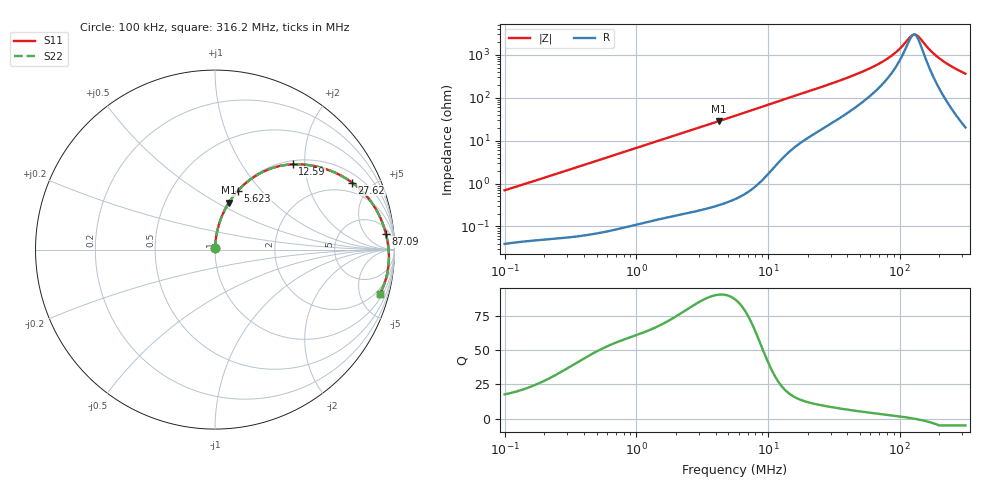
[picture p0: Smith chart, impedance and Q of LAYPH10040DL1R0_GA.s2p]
! LAYPH10040DL1R0_GA  S-PARAMETER MODEL  ( General Type )
! Model Generated by TAIYO YUDEN Corporation (http://www.ty-top.com)
! Version 1.0
! TAIYO YUDEN Control No. 180920NI43SB-FBB
! Copyright(c) 2018 TAIYO YUDEN CO.,LTD. All Rights Reserved.
! Product Description (link to TY-COMPAS)
! https://ds.yuden.co.jp/TYCOMPAS/or/detail?pn=LAYPH10040DL1R0NGA&u=M
! Products Name : Inductors
! Characteristics :
!  Inductance : 1 uH , SRF(min) : -Hz , DC Resistance(max) : 0.01 Ohm
!  Rated Current : Saturation :10.7 A , Temp Rise : 3.6 A (25 degC)
!  Case Size : 10.1 x 10.0 / 0.398 x 0.394 [mm/inch] , Thickness : 4 / 0.157 [mm/inch]
!  (Conditions: Temperature = 25 degC , DC Bias Current/Voltage = 0A / 0V)
! External Node Assignments :
!  1  o---GGG---o  2
! GND o---------o GND
! Frequency Range : 0.1MHz  -  316.199832MHz  [ 402 STEP ]
# MHz S RI R 50
! Freq[MHz].  S11 Real  S11 Imag  S21 Real  S21 Imag  S12 Real  S12 Imag  S22 Real  S22 Imag
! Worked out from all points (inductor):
!   401 points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, 100 kHz to 316.2 MHz, reference 50 ohm
!   read as one part in series: L = 1.09 uH near 104.1 kHz
!   highest Q = 90.7 at 4.241 MHz (marker M1), where L = 1.06 uH
!   self-resonance near 128.5 MHz
!   S11 on the Smith chart (normalised r, x): 100 kHz: 1.00, +0.01; 5.623 MHz: 1.01, +0.75; 12.59 MHz: 1.07, +1.73; 27.62 MHz: 1.42, +3.83; 87.09 MHz: 8, +17; 316.2 MHz: 1.41, -7.23
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0.1  0.00044 0.00694  0.9996 -0.00694  0.9996 -0.00694  0.00044 0.00694
0.385695  0.00129 0.026  0.9987 -0.026  0.9987 -0.026  0.00129 0.026
1.487603  0.0113 0.0984  0.9887 -0.0984  0.9887 -0.0984  0.0113 0.0984
2.562917  0.0304 0.1657  0.9696 -0.1657  0.9696 -0.1657  0.0304 0.1657
4.241136  0.0769 0.261  0.9231 -0.261  0.9231 -0.261  0.0769 0.261
5.623165  0.1274 0.3277  0.8726 -0.3277  0.8726 -0.3277  0.1274 0.3277
8.245728  0.2416 0.4199  0.7584 -0.4199  0.7584 -0.4199  0.2416 0.4199
12.58859  0.4324 0.4752  0.5676 -0.4752  0.5676 -0.4752  0.4324 0.4752
21.68824  0.6777 0.4248  0.3223 -0.4248  0.3223 -0.4248  0.6777 0.4248
27.61997  0.7641 0.3732  0.2359 -0.3732  0.2359 -0.3732  0.7641 0.3732
53.69948  0.9087 0.2033  0.0913 -0.2033  0.0913 -0.2033  0.9087 0.2033
68.38627  0.9347 0.1444  0.0653 -0.1444  0.0653 -0.1444  0.9347 0.1444
83.65039  0.9497 0.0977  0.0503 -0.0977  0.0503 -0.0977  0.9497 0.0977
87.0899  0.9521 0.0885  0.0479 -0.0885  0.0479 -0.0885  0.9521 0.0885
100.2806  0.9592 0.0566  0.0408 -0.0566  0.0408 -0.0566  0.9592 0.0566
122.6637  0.9662 0.0107  0.0338 -0.0107  0.0338 -0.0107  0.9662 0.0107
132.9584  0.9678 -0.00807  0.0322 0.00807  0.0322 0.00807  0.9678 -0.00807
141.2425  0.9686 -0.0224  0.0314 0.0224  0.0314 0.0224  0.9686 -0.0224
172.7685  0.9681 -0.0726  0.0319 0.0726  0.0319 0.0726  0.9681 -0.0726
198.9362  0.9639 -0.1102  0.0361 0.1102  0.0361 0.1102  0.9639 -0.1102
248.292  0.9491 -0.174  0.0509 0.174  0.0509 0.174  0.9491 -0.174
316.1998  0.917 -0.2492  0.083 0.2492  0.083 0.2492  0.917 -0.2492
